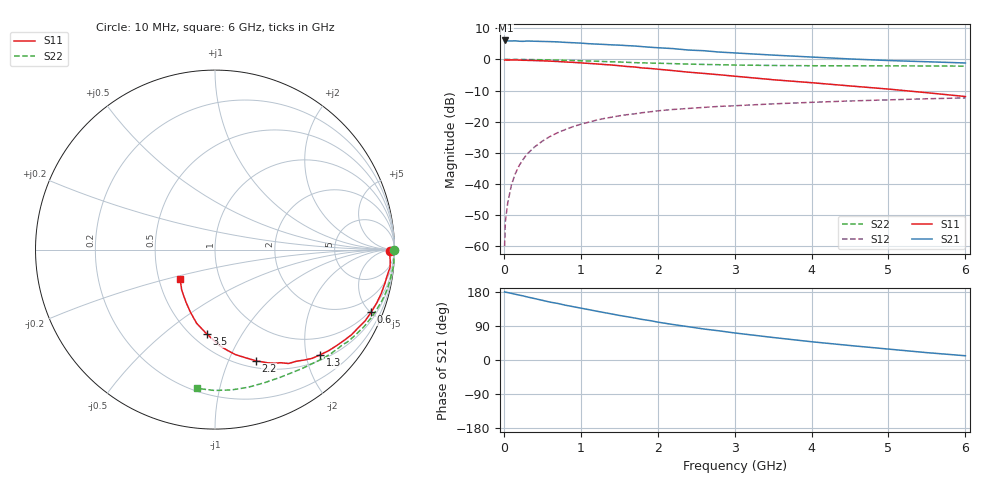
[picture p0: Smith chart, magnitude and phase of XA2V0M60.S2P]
! SIEMENS Discrete & RF Semiconductors
! BFY180
! Si NPN RF Bipolar Junction Transistor in MICRO-X
! VCE = 2 V  IC = 0.6 mA
! Common Emitter S-Parameters:  May  1997
# GHz  S  MA  R  50
!  f  S11  S21  S12  S22
! GHz  MAG  ANG  MAG  ANG  MAG  ANG  MAG  ANG
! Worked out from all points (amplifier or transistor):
!   36 points, 10 MHz to 6 GHz, reference 50 ohm
!   highest |S21| = 6.1 dB at 20 MHz (marker M1)
!   |S21| within 3 dB of that: start of sweep to 2.365 GHz
!   unconditionally stable (mu >= 1): 4.613 GHz to end of sweep
!   at 250 MHz: K = 0.06, MSG = 19.0 dB, |S12| = -32.1 dB
!   at 1.4 GHz: K = 0.43, MSG = 11.6 dB, |S12| = -18.6 dB
!   at 6 GHz: K = 1.04, MAG = 4.4 dB, |S12| = -12.4 dB
!   S11 on the Smith chart (normalised r, x): 10 MHz: 78, -17; 600 MHz: 0.88, -5.05; 1.3 GHz: 0.61, -2.27; 2.2 GHz: 0.58, -1.26; 3.5 GHz: 0.59, -0.71; 6 GHz: 0.64, -0.22
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0.01  0.9759 -0.3  1.964 179.8  0.001 106.0  0.9983 -0.2
0.02  0.9778 -0.6  2.015 179.0  0.0025 84.3  0.9999 -0.5
0.05  0.9739 -1.6  1.983 178.0  0.0049 84.2  0.9989 -1.2
0.1  0.9782 -3.6  1.979 175.8  0.0098 86.9  0.9967 -2.4
0.15  0.9805 -5.9  1.986 173.5  0.0147 85.6  0.9993 -3.6
0.2  0.9744 -7.3  1.958 171.2  0.0198 85.4  0.9969 -4.8
0.3  0.9657 -11.0  1.974 166.6  0.03 81.9  0.9936 -7.2
0.4  0.9582 -14.7  1.958 162.1  0.0393 79.1  0.9911 -9.5
0.6  0.9376 -21.8  1.93 152.8  0.0578 73.6  0.9813 -14.2
0.8  0.9084 -28.8  1.877 144.6  0.0748 68.4  0.9665 -18.7
1.1  0.8627 -38.4  1.788 133.1  0.0978 60.9  0.9428 -25.1
1.3  0.8283 -45.1  1.741 125.3  0.1122 56.1  0.9249 -29.2
1.5  0.7916 -51.0  1.695 117.7  0.124 51.9  0.9077 -33.1
1.7  0.7558 -57.1  1.642 110.8  0.1335 48.1  0.8865 -36.7
2.2  0.6599 -69.8  1.491 93.6  0.1569 39.6  0.8553 -45.1
2.6  0.5951 -79.1  1.379 81.8  0.1694 34.3  0.8302 -50.9
3  0.5374 -87.0  1.271 71.4  0.1801 29.3  0.8124 -56.6
3.5  0.4716 -95.7  1.172 59.4  0.1931 24.5  0.799 -63.0
4  0.4225 -104.1  1.091 48.2  0.2043 19.4  0.7912 -69.6
4.5  0.3748 -111.4  1.017 38.2  0.215 15.0  0.789 -76.3
5.5  0.2916 -129.5  0.917 19.4  0.2331 6.4  0.7848 -90.2
6  0.2534 -140.3  0.876 11.2  0.2408 1.9  0.7797 -97.2
